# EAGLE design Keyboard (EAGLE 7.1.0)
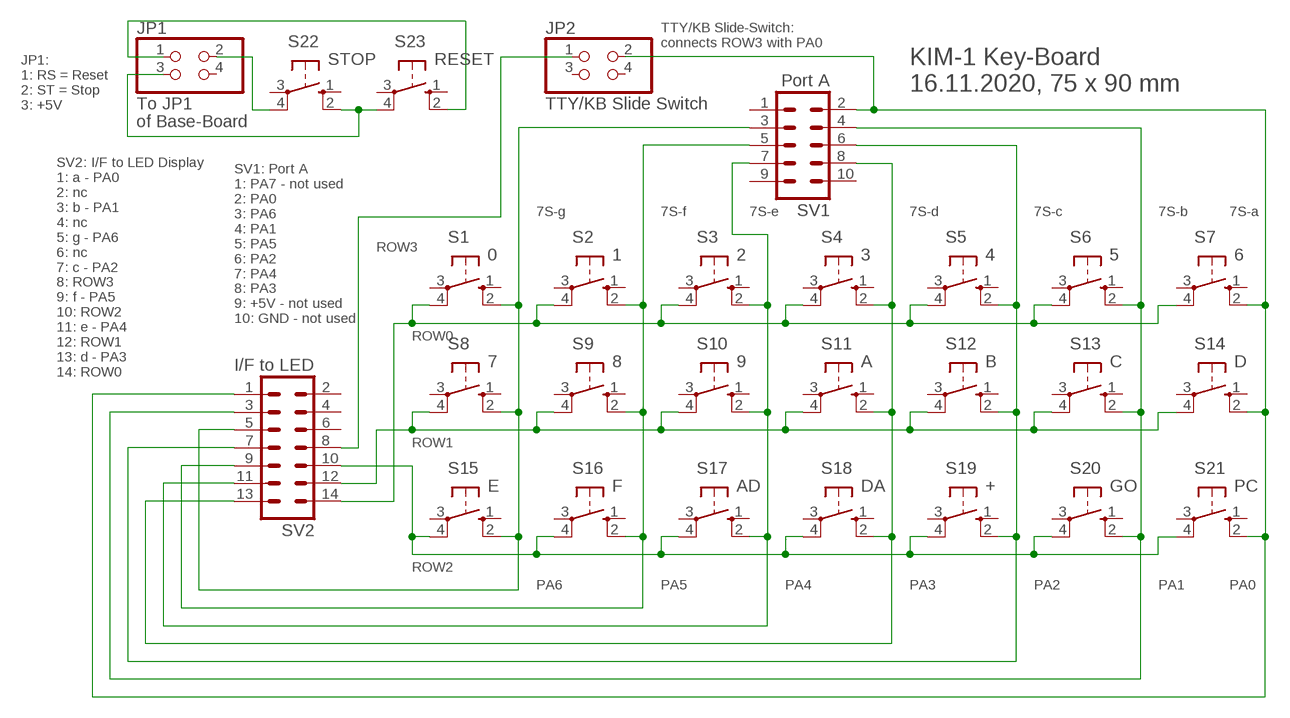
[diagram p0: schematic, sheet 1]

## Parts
JP1  To JP1  PINHD-2X2  [2X02]
JP2  TTY/KB Slide Switch  PINHD-2X2  [2X02]
S1  0  10-XX  [B3F-10XX]
S2  1  10-XX  [B3F-10XX]
S3  2  10-XX  [B3F-10XX]
S4  3  10-XX  [B3F-10XX]
S5  4  10-XX  [B3F-10XX]
S6  5  10-XX  [B3F-10XX]
S7  6  10-XX  [B3F-10XX]
S8  7  10-XX  [B3F-10XX]
S9  8  10-XX  [B3F-10XX]
S10  9  10-XX  [B3F-10XX]
S11  A  10-XX  [B3F-10XX]
S12  B  10-XX  [B3F-10XX]
S13  C  10-XX  [B3F-10XX]
S14  D  10-XX  [B3F-10XX]
S15  E  10-XX  [B3F-10XX]
S16  F  10-XX  [B3F-10XX]
S17  AD  10-XX  [B3F-10XX]
S18  DA  10-XX  [B3F-10XX]
S19  +  10-XX  [B3F-10XX]
S20  GO  10-XX  [B3F-10XX]
S21  PC  10-XX  [B3F-10XX]
S22  STOP  10-XX  [B3F-10XX]
S23  RESET  10-XX  [B3F-10XX]
SV1  Port A  ML10  [ML10]
SV2  I/F to LED  ML14  [ML14]

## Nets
N$1: S8.4(P1) S9.4(P1) S10.4(P1) S11.4(P1) S12.4(P1) S13.4(P1) S14.4(P1) SV2.12
N$2: JP1.3 S22.2(S1) S23.4(P1)
N$3: JP2.2 S7.2(S1) S14.2(S1) S21.2(S1) SV1.2 SV2.1
N$5: S5.2(S1) S12.2(S1) S19.2(S1) SV1.6 SV2.7
N$6: S4.2(S1) S11.2(S1) S18.2(S1) SV1.8 SV2.13
N$7: S3.2(S1) S10.2(S1) S17.2(S1) SV1.7 SV2.11
N$8: S2.2(S1) S9.2(S1) S16.2(S1) SV1.5 SV2.9
N$9: S1.2(S1) S8.2(S1) S15.2(S1) SV1.3 SV2.5
N$10: S15.4(P1) S16.4(P1) S17.4(P1) S18.4(P1) S19.4(P1) S20.4(P1) S21.4(P1) SV2.10
N$11: S1.4(P1) S2.4(P1) S3.4(P1) S4.4(P1) S5.4(P1) S6.4(P1) S7.4(P1) SV2.14
N$12: JP1.1 S23.2(S1)
N$13: JP1.2 S22.4(P1)
N$16: JP2.1 SV2.8
N$21: S6.2(S1) S13.2(S1) S20.2(S1) SV1.4 SV2.3
Unconnected: JP1.4 JP2.3 JP2.4 S1.1(S) S1.3(P) S2.1(S) S2.3(P) S3.1(S) S3.3(P) S4.1(S) S4.3(P) S5.1(S) S5.3(P) S6.1(S) S6.3(P) S7.1(S) S7.3(P) S8.1(S) S8.3(P) S9.1(S) S9.3(P) S10.1(S) S10.3(P) S11.1(S) S11.3(P) S12.1(S) S12.3(P) S13.1(S) S13.3(P) S14.1(S) S14.3(P) S15.1(S) S15.3(P) S16.1(S) S16.3(P) S17.1(S) S17.3(P) S18.1(S) S18.3(P) S19.1(S) S19.3(P) S20.1(S) S20.3(P) S21.1(S) S21.3(P) S22.1(S) S22.3(P) S23.1(S) S23.3(P) SV1.1 SV1.9 SV1.10 SV2.2 SV2.4 SV2.6

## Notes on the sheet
- TTY/KB Slide-Switch:
  connects ROW3 with PA0
- KIM-1 Key-Board
  16.11.2020, 75 x 90 mm
- JP1:
  1: RS = Reset
  2: ST = Stop
  3: +5V
- of Base-Board
- 7S-g | 7S-f | 7S-e | 7S-d | 7S-c | 7S-b | 7S-a
- ROW3
- SV1: Port A
  1: PA7 - not used
  2: PA0
  3: PA6
  4: PA1
  5: PA5
  6: PA2
  7: PA4
  8: PA3
  9: +5V - not used
  10: GND - not used
- ROW0
- SV2: I/F to LED Display
  1: a - PA0
  2: nc
  3: b - PA1
  4: nc
  5: g - PA6
  6: nc
  7: c - PA2
  8: ROW3
  9: f - PA5
  10: ROW2
  11: e - PA4
  12: ROW1
  13: d - PA3
  14: ROW0
- ROW1
- ROW2
- PA6 | PA5 | PA4 | PA3 | PA2 | PA1 | PA0

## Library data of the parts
JP1 JP2 = 11manni:PINHD-2X2: PIN HEADER
S1-S23 = switch-omron:10-XX: OMRON SWITCH; MPN: B3F-1000; OC_FARNELL: 176432; OC_NEWARK: 36M3542
SV1 = con-harting-ml:ML10: HARTING; OC_FARNELL: unknown; OC_NEWARK: unknown
SV2 = con-harting-ml:ML14: HARTING; OC_FARNELL: unknown; OC_NEWARK: unknown

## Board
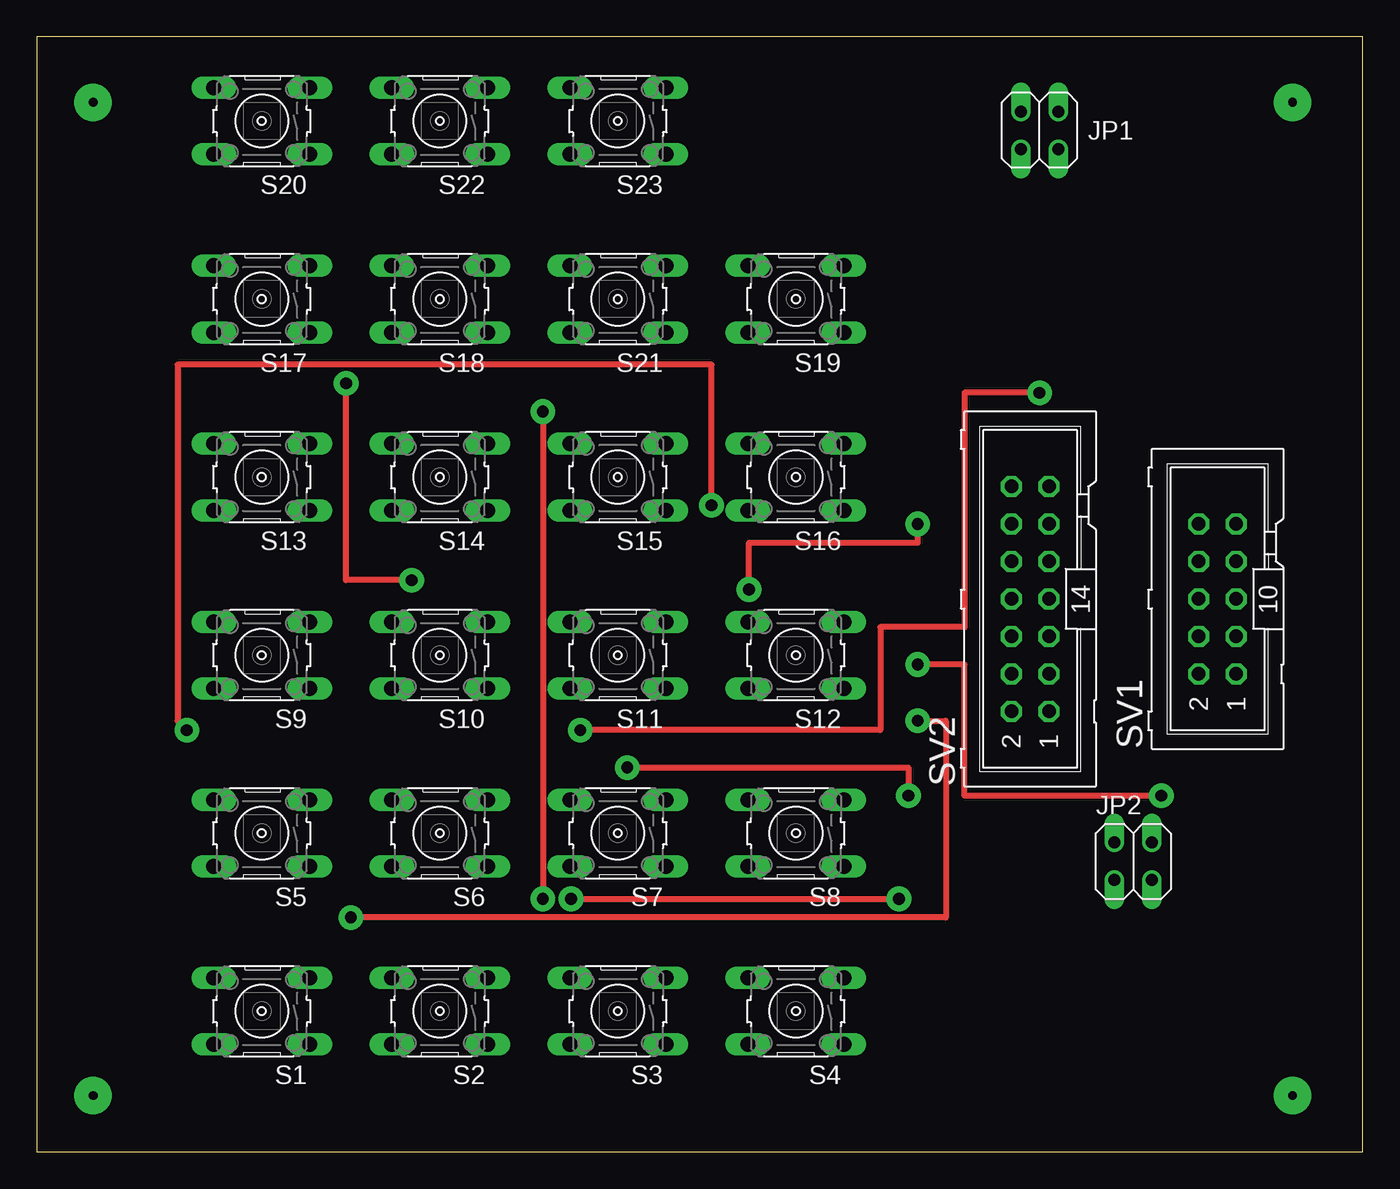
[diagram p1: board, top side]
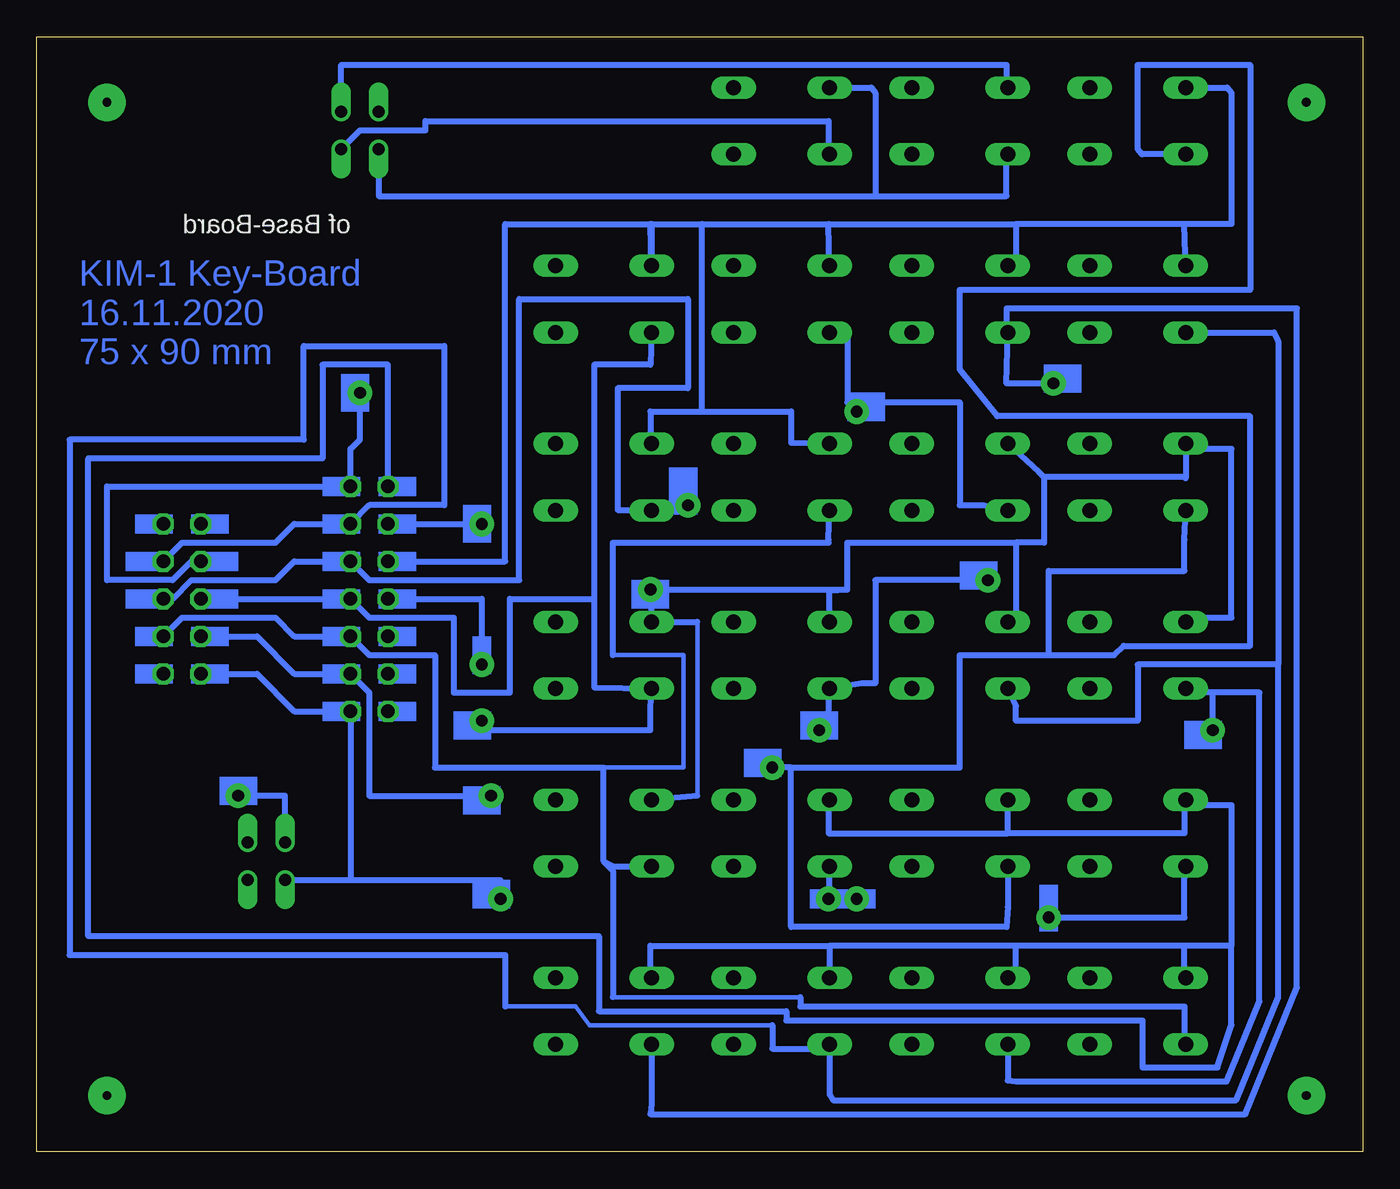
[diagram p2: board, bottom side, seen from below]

Size 89.84 x 75.56 mm. Coordinates in mm from the lower left corner, seen from the top.
Outline: 0,0 89.84,0 89.84,75.56 0,75.56 0,0
Copper layers (1*16): Top 0.035mm / dielectric 1.5mm / Bottom 0.035mm
Design rules "default": minimum track width 10mil, minimum drill 24mil, track to track 8mil, track to pad 8mil, pad to pad 8mil, via to via 8mil, smd to smd 8mil, copper to edge 40mil, drill to drill 8mil, minimum pad ring 10mil, minimum via ring 8mil, stop-mask expansion 4mil, vias tented up to drill 0mil, thermal gap 10mil

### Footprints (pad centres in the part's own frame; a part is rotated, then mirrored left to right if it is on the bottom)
2X02 = drill 0.8 offset: 1 -1.27,1.27; 2 -1.27,-1.27; 3 1.27,1.27; 4 1.27,-1.27
B3F-10XX = drill 1.016 long: 1 -3.251,2.261; 2 3.251,2.261; 3 -3.251,-2.261; 4 3.251,-2.261
ML10 = drill 0.914 octagon: 1 -5.08,-1.27; 2 -5.08,1.27; 3 -2.54,-1.27; 4 -2.54,1.27; 5 0,-1.27; 6 0,1.27; 7 2.54,-1.27; 8 2.54,1.27; 9 5.08,-1.27; 10 5.08,1.27
ML14 = drill 0.914 octagon: 1 -7.62,-1.27; 2 -7.62,1.27; 3 -5.08,-1.27; 4 -5.08,1.27; 5 -2.54,-1.27; 6 -2.54,1.27; 7 0,-1.27; 8 0,1.27; 9 2.54,-1.27; 10 2.54,1.27; 11 5.08,-1.27; 12 5.08,1.27; 13 7.62,-1.27; 14 7.62,1.27

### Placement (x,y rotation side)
JP1  67.94,69.22 180 top
JP2  74.3,19.68 0 top
S1  15.24,9.53 180 top
S2  27.3,9.53 180 top
S3  39.37,9.53 180 top
S4  51.44,9.53 180 top
S5  15.24,21.59 180 top
S6  27.3,21.59 180 top
S7  39.37,21.59 180 top
S8  51.44,21.59 180 top
S9  15.24,33.66 180 top
S10  27.3,33.66 180 top
S11  39.37,33.66 180 top
S12  51.44,33.66 180 top
S13  15.24,45.72 180 top
S14  27.3,45.72 180 top
S15  39.37,45.72 180 top
S16  51.44,45.72 180 top
S17  15.24,57.78 180 top
S18  27.3,57.78 180 top
S19  51.44,57.78 180 top
S20  15.24,69.85 180 top
S21  39.37,57.78 180 top
S22  27.3,69.85 180 top
S23  39.37,69.85 180 top
SV1  80.01,37.47 90 top
SV2  67.31,37.47 90 top

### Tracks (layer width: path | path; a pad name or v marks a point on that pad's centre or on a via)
N$1  (via drill 0.8 pad 1.68)
  Top 0.406: v48.26,38.1 48.26,41.27 59.69,41.27 v59.69,42.55
  Bottom 0.305: 45.09,35.92 45.09,24.13
  Bottom 0.406: 21.59,45.72 12.06,45.72 11.99,45.64 S13.4 11.71,47.62 8.89,47.62 8.89,36.2 12.06,36.2 11.99,36.12 S9.4 | 24.13,48.06 S14.4 21.95,46.08 21.59,45.72 | 21.59,45.72 21.59,41.27 23.5,41.27 | 23.5,41.27 23.5,35.99 S10.4 | S11.4 36.12,38.02 34.92,38.1 | 34.92,38.1 34.92,41.27 23.5,41.27 | 34.92,38.1 v48.26,38.1 48.18,37.39 S12.4 45.09,35.92 | 45.09,24.13 S8.4 | SV2.12 v59.69,42.55
N$2
  Bottom 0.305: 24.13,67.51 S22.2
  Bottom 0.406: JP1.3 66.67,64.77 33.02,64.77 | 33.02,64.77 24.13,64.77 24.13,67.51 | S23.4 33.3,72.11 33.02,71.75 33.02,64.77
N$3  (via drill 0.8 pad 1.68)
  Top 0.406: v34.29,50.16 v34.29,17.14 | v36.2,17.14 v58.42,17.14
  Bottom 0.406: SV1.2 74.93,32.38 72.39,29.84 SV2.1 68.58,18.41 | S21.2 34.92,55.52 34.92,50.8 34.29,50.8 | 34.29,50.8 27.3,50.8 27.3,43.81 25.68,43.81 S14.2 | 34.57,17.14 v34.29,17.14 v36.2,17.14 36.12,17.14 S7.2 | v34.29,50.16 34.29,50.8 | v58.42,17.14 58.42,18.41 68.58,18.41 | JP2.2 68.58,18.41
N$5  (via drill 0.8 pad 1.68)
  Top 0.406: v59.69,29.21 61.59,29.21 61.59,15.88 v21.27,15.88
  Bottom 0.406: SV1.6 SV2.7 67.31,36.2 61.59,36.2 61.59,31.11 57.78,31.11 57.78,37.47 52.07,37.47 | S19.2 48.26,53.34 52.07,53.34 52.07,37.47 | 52.07,37.47 52.07,31.47 S12.2 48.26,30.05 48.26,28.57 59.69,28.57 v59.69,29.21 | v21.27,15.88 12.06,15.88 12.06,18.62 | 12.06,18.73 12.06,18.62 | 12.06,18.62 S5.2
N$6  (via drill 0.8 pad 1.68)
  Top 0.406: v25.4,38.73 20.95,38.73 v20.95,52.07 | v67.94,51.44 62.87,51.44 62.87,35.56 57.15,35.56 57.15,28.57 v36.83,28.57
  Bottom 0.406: SV1.8 79.38,40.01 80.64,38.73 85.09,38.73 85.09,45.09 SV2.13 68.58,47.62 67.94,48.26 v67.94,51.44 | S4.2 48.18,3.25 48.26,2.54 7.94,2.54 4.45,11.11 4.45,57.15 24.13,57.15 24.13,56.24 S18.2 24.13,52.07 v20.95,52.07 | v25.4,38.73 33.02,38.73 33.02,31.75 33.93,31.75 S11.2 36.2,29.41 v36.83,28.57
N$7
  Bottom 0.305: 58.1,9.84 53.34,9.84 52.39,8.57 40.01,8.57
  Bottom 0.406: SV1.7 80.01,41.27 73.66,41.27 72.39,42.55 SV2.11 67.31,43.81 62.23,43.81 62.23,54.61 71.75,54.61 71.75,48.26 87.63,48.26 87.63,13.34 58.1,13.34 58.1,9.84 | 5.71,33.02 5.71,10.48 8.57,3.49 35.88,3.49 36.12,3.89 S3.2 36.4,6.99 40.01,6.99 40.01,8.57 | 5.71,33.02 15.24,33.02 15.24,29.21 23.5,29.21 23.5,30.2 S10.2 | S17.2 5.99,55.52 5.71,54.93 5.71,33.02
N$8  (via drill 0.8 pad 1.68)
  Top 0.406: v45.72,43.81 45.72,53.34 9.53,53.34 9.53,29.21 v10.16,28.57
  Bottom 0.406: SV1.5 80.64,37.47 79.38,38.73 73.66,38.73 72.39,40.01 SV2.9 67.31,38.73 57.15,38.73 57.15,57.78 45.72,57.78 45.72,51.75 50.48,51.75 50.48,43.5 48.18,43.5 S16.2 48.26,43.54 48.26,43.81 v45.72,43.81 | S2.2 24.05,4.84 23.5,4.76 9.21,4.76 6.99,10.16 6.99,31.11 10.16,31.11 | 10.16,31.11 11.71,31.11 S9.2 | v10.16,28.57 10.16,31.11
N$9
  Bottom 0.305: 50.8,10.48 38.1,10.48 | 51.44,26.04 46.04,26.04 46.04,33.66 50.8,33.66
  Bottom 0.406: SV1.3 80.01,36.2 73.66,36.2 72.39,34.92 SV2.5 67.31,33.66 62.87,33.66 62.87,26.04 51.44,26.04 51.44,19.68 | 51.44,19.68 50.8,19.05 50.8,10.48 | 38.1,10.48 38.1,9.84 12.06,9.84 12.06,7.34 S1.2 | 51.44,19.68 50.76,19.33 S8.2 | 50.8,33.66 50.8,41.27 36.2,41.27 36.2,41.48 S15.2
N$10
  Bottom 0.406: S20.4 9.17,72.11 8.89,71.75 8.89,62.87 12.06,62.87 | S17.4 11.99,59.77 12.06,62.87 | 12.06,62.87 23.5,62.87 | 23.5,62.87 23.5,59.97 S18.4 | S21.4 36.12,59.77 36.2,62.87 | 36.2,62.87 23.5,62.87 | 48.26,62.87 48.18,59.77 S19.4 48.18,62.87 | 48.26,62.87 48.18,62.87 | 48.18,62.87 44.77,62.87 | 44.77,62.87 36.2,62.87 | 44.77,50.16 44.77,62.87 | 44.77,50.16 38.73,50.16 38.73,48.06 S15.4 | 44.77,50.16 48.26,50.16 48.26,48.06 S16.4 | SV2.10 58.1,40.01 58.1,62.87 48.26,62.87
N$11
  Bottom 0.406: 8.89,13.97 8.89,23.5 11.99,23.5 S5.4 12.06,23.22 12.06,21.59 24.05,21.59 | 24.05,21.59 S6.4 | S7.4 36.2,23.22 36.2,21.59 24.05,21.59 | S4.4 48.26,11.79 48.26,13.97 36.12,13.97 | 36.12,13.97 S3.4 | S2.4 23.5,11.79 23.5,13.97 | 23.5,13.97 36.12,13.97 | S1.4 12.06,11.79 12.06,13.97 | 12.06,13.97 23.5,13.97 | 8.89,13.97 12.06,13.97 | SV2.14 66.04,53.34 70.48,53.34 70.48,46.99 86.36,46.99 86.36,14.61 51.75,14.61 51.75,9.53 39.05,9.53 39.05,8.89 14.92,8.89 14.92,5.71 9.84,5.71 8.89,8.57 8.89,13.97
N$12
  Bottom 0.406: JP1.1 67.94,69.22 63.5,69.22 63.5,69.85 36.2,69.85 36.2,67.03 S23.2
N$13
  Bottom 0.406: JP1.2 69.22,73.66 24.13,73.66 24.13,72.19 S22.4
N$16  (via drill 0.8 pad 1.68)
  Top 0.406: v76.2,24.13 62.87,24.13 62.87,33.02 v59.69,33.02
  Bottom 0.406: SV2.8 59.69,37.47 v59.69,33.02 | JP2.1 73.03,24.13 v76.2,24.13
N$17  (via drill 0.6 pad 2.54)
  other vias: 3.81,71.12
N$18  (via drill 0.6 pad 2.54)
  other vias: 85.09,71.12
N$19  (via drill 0.6 pad 2.54)
  other vias: 3.81,3.81
N$20  (via drill 0.6 pad 2.54)
  other vias: 85.09,3.81
N$21  (via drill 0.8 pad 1.68)
  Top 0.406: v40.01,26.04 59.05,26.04 v59.05,24.13
  Bottom 0.406: 21.27,33.66 16.83,33.66 16.19,34.29 7.62,34.29 7.62,49.85 24.77,49.85 27.3,53.02 27.3,58.42 7.62,58.42 7.62,73.66 15.24,73.66 15.24,67.94 14.96,67.59 S20.2 | SV1.4 74.93,34.92 72.39,32.38 SV2.3 67.31,31.11 67.31,24.13 v59.05,24.13 | S6.2 24.05,16.59 24.13,15.24 38.73,15.24 38.73,26.04 | 38.73,26.04 27.3,26.04 27.3,33.66 21.27,33.66 | 21.27,33.66 21.27,39.37 12.06,39.37 12.06,41.48 S13.2 | 38.73,26.04 v40.01,26.04
(copper drawn outside any net)
  shapes: Bottom area x41

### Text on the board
Bottom: KIM-1 Key-Board / 16.11.2020 / 75 x 90 mm
bNames: of Base-Board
